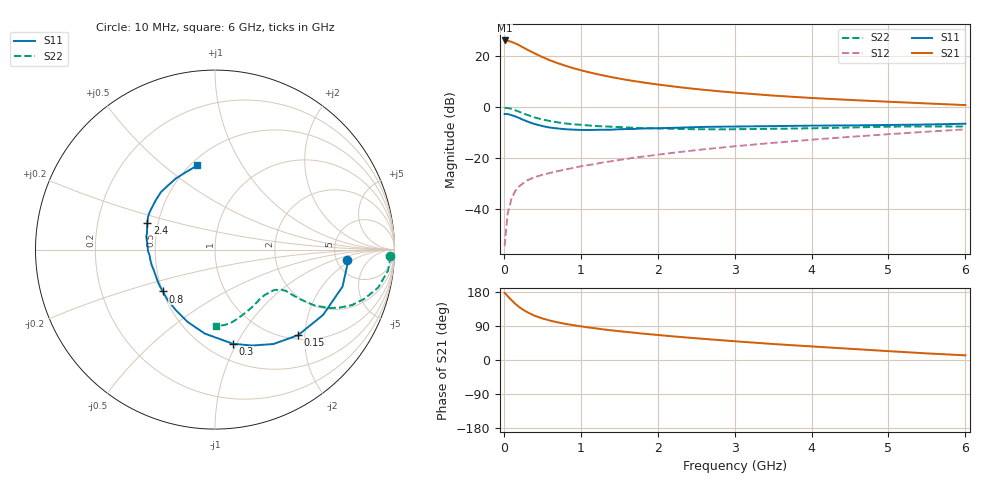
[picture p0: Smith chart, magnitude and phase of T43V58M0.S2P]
! Infineon Technologies  Discrete & RF Semiconductors
! BFR182T
! Si NPN RF Bipolar Junction Transistor in SC75
! VCE = 3.5 V  IC = 8 mA
! Common Emitter S-Parameters:  October  1999
# GHz  S  MA  R  50
!  f  S11  S21  S12  S22
! GHz  MAG  ANG  MAG  ANG  MAG  ANG  MAG  ANG
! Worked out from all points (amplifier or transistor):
!   36 points, 10 MHz to 6 GHz, reference 50 ohm
!   highest |S21| = 26.3 dB at 10 MHz (marker M1)
!   |S21| within 3 dB of that: start of sweep to 267.6 MHz
!   unconditionally stable (mu >= 1): 1.121 GHz to 3.862 GHz
!   at 250 MHz: K = 0.39, MSG = 26.7 dB, |S12| = -29.8 dB
!   at 1.4 GHz: K = 1.06, MAG = 15.0 dB, |S12| = -21.1 dB
!   at 6 GHz: K = 0.84, MSG = 4.8 dB, |S12| = -8.6 dB
!   lowest NFmin = 1.40 dB at 450 MHz
!   S11 on the Smith chart (normalised r, x): 10 MHz: 6.31, -1.55; 150 MHz: 1.08, -1.85; 300 MHz: 0.66, -0.96; 800 MHz: 0.50, -0.27; 2.4 GHz: 0.44, +0.16; 6 GHz: 0.54, +0.66
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0.01  0.7402 -4.3  20.57 176.7  0.0019 79.6  0.9767 -2.1
0.02  0.7443 -5.2  20.39 175.5  0.0028 95.7  0.9783 -2.6
0.05  0.7398 -16.2  20.3 168.4  0.0083 86.5  0.9712 -6.9
0.1  0.7037 -31.1  19.3 157.9  0.0163 76.5  0.9333 -13.1
0.15  0.6648 -45.8  17.99 148.0  0.0232 69.8  0.8769 -18.2
0.2  0.6188 -58.2  16.55 139.7  0.0283 66.8  0.8224 -22.1
0.25  0.5727 -69.0  15.05 132.7  0.0325 62.2  0.765 -25.0
0.3  0.5333 -79.4  13.7 126.6  0.0369 60.7  0.7178 -27.0
0.4  0.4715 -96.9  11.46 116.8  0.0429 57.2  0.6362 -29.3
0.5  0.4312 -110.6  9.734 109.8  0.0476 56.2  0.5807 -29.9
0.6  0.4024 -122.5  8.39 104.0  0.0519 56.5  0.5396 -30.3
0.7  0.3865 -132.5  7.38 99.4  0.0563 57.5  0.5085 -30.3
0.8  0.3732 -141.3  6.573 95.3  0.0605 57.9  0.4857 -30.4
1.1  0.3598 -161.7  4.921 85.8  0.0741 60.6  0.4428 -30.8
1.3  0.3648 -171.3  4.218 80.6  0.0842 61.9  0.4239 -31.8
1.6  0.3764 177.2  3.463 73.9  0.0983 63.2  0.4045 -33.6
2.2  0.3977 162.0  2.578 62.4  0.1289 64.6  0.3818 -39.7
2.4  0.4062 158.2  2.378 59.0  0.1396 65.0  0.3753 -42.2
3.5  0.4298 140.0  1.706 42.2  0.2017 63.0  0.3809 -56.6
4.5  0.4428 126.4  1.401 29.6  0.2647 59.1  0.4035 -71.2
5.5  0.4622 109.9  1.197 17.4  0.3341 53.9  0.4243 -84.0
6  0.4789 101.8  1.111 12.3  0.3712 50.3  0.4238 -89.3
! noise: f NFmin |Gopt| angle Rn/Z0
0.45  1.4  0.26  41  0.29
0.9  1.5  0.25  83  0.23
1.8  2  0.21  162  0.2
